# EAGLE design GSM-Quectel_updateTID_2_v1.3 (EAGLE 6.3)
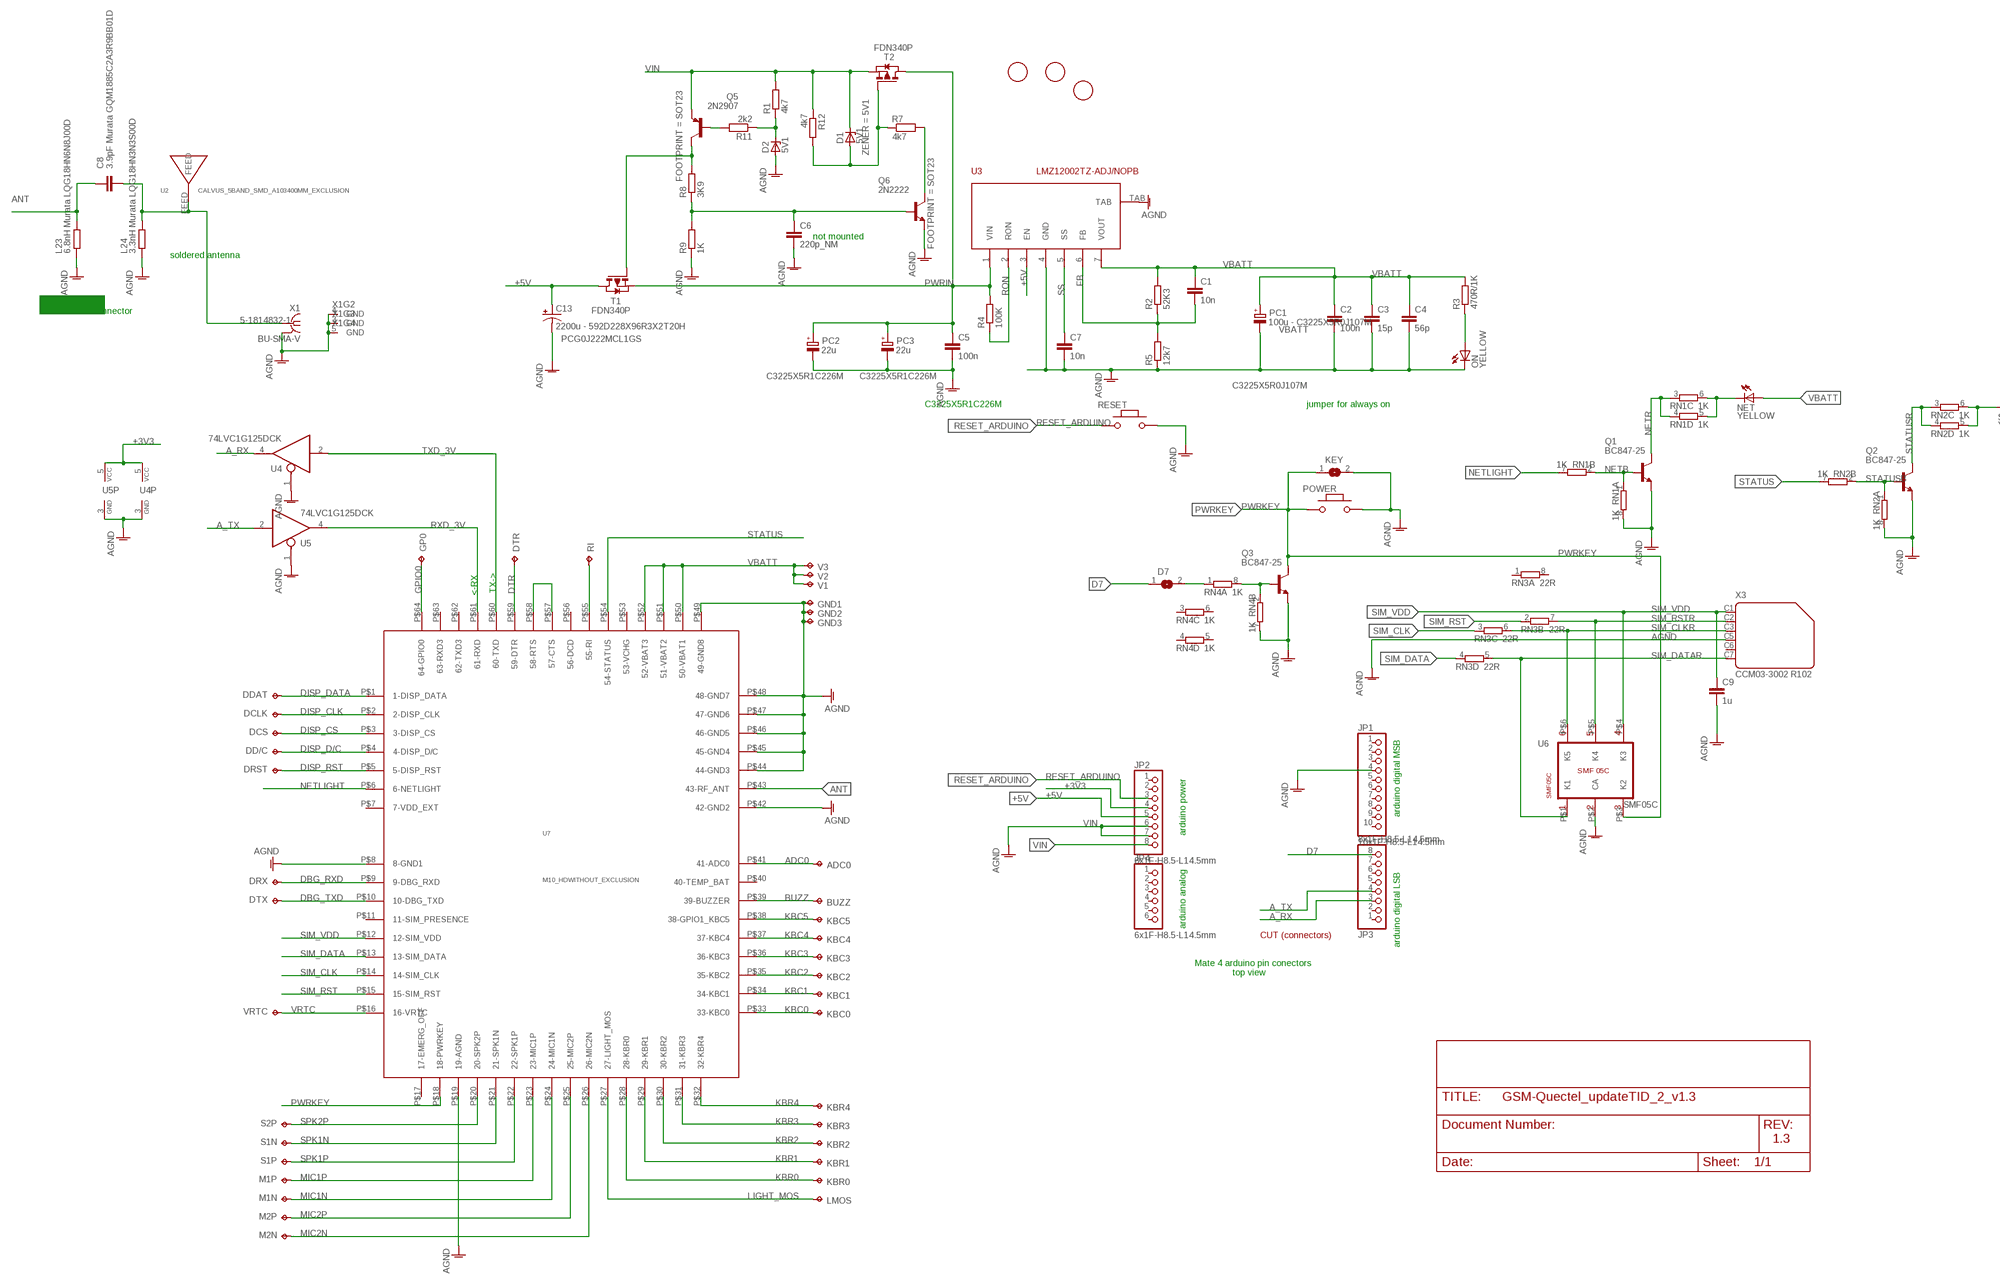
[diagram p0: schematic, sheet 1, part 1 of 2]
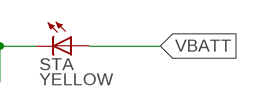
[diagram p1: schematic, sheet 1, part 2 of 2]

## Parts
ADC0  TPPAD1-09  [P1-09]
BUZZ  TPPAD1-09  [P1-09]
C1  10n  C-EU0603-RND  [C0603-ROUND]
C2  100n  C-EU0603-RND  [C0603-ROUND]
C3  15p  C-EU0603-RND  [C0603-ROUND]
C4  56p  C-EU0603-RND  [C0603-ROUND]
C5  100n  C-EU0603-RND  [C0603-ROUND]
C6  220p_NM  C-EU0603-RND  [C0603-ROUND]
C7  10n  C-EU0603-RND  [C0603-ROUND]
C8  3.9pF Murata GQM1885C2A3R9BB01D  C-EU0603-RND  [C0603-ROUND]
C9  1u  C-EU0603-RND  [C0603-ROUND]
C13  2200u - 592D228X96R3X2T20H  CPOL-US085CS-1AW  [085CS_1AW]
D1  5V1  ZENER-DIODESMB  [SMB]
D2  5V1  ZENER-DIODESMB  [SMB]
D7  SJ  [SJ]
DCLK  TPPAD1-09  [P1-09]
DCS  TPPAD1-09  [P1-09]
DD/C  TPPAD1-09  [P1-09]
DDAT  TPPAD1-09  [P1-09]
DRST  TPPAD1-09  [P1-09]
DRX  TPPAD1-09  [P1-09]
DTR  TPPAD1-09  [P1-09]
DTX  TPPAD1-09  [P1-09]
GND1  TPPAD1-09  [P1-09]
GND2  TPPAD1-09  [P1-09]
GND3  TPPAD1-09  [P1-09]
GP0  TPPAD1-09  [P1-09]
JP1  10x1F-H8.5-L14.5mm  PINHD-1X10TH  [1X10-TH]
JP2  8x1F-H8.5-L14.5mm  PINHD-1X8TH  [1X08-TH]
JP3  8x1F-H8.5-L14.5mm  PINHD-1X8TH  [1X08-TH]
JP4  6x1F-H8.5-L14.5mm  PINHD-1X6TH  [1X06-TH]
KBC0  TPPAD1-09  [P1-09]
KBC1  TPPAD1-09  [P1-09]
KBC2  TPPAD1-09  [P1-09]
KBC3  TPPAD1-09  [P1-09]
KBC4  TPPAD1-09  [P1-09]
KBC5  TPPAD1-09  [P1-09]
KBR0  TPPAD1-09  [P1-09]
KBR1  TPPAD1-09  [P1-09]
KBR2  TPPAD1-09  [P1-09]
KBR3  TPPAD1-09  [P1-09]
KBR4  TPPAD1-09  [P1-09]
KEY  SJ  [SJ]
L23  6.8nH Murata LQG18HN6N8J00D  R-EU_0603-RND  [R0603-ROUND]
L24  3.3nH Murata LQG18HN3N3S00D  R-EU_0603-RND  [R0603-ROUND]
LMOS  TPPAD1-09  [P1-09]
M1N  TPPAD1-09  [P1-09]
M1P  TPPAD1-09  [P1-09]
M2N  TPPAD1-09  [P1-09]
M2P  TPPAD1-09  [P1-09]
NET  YELLOW  LEDCHIP-LED0805  [CHIP-LED0805]
ON  YELLOW  LEDCHIP-LED0805  [CHIP-LED0805]
PC1  100u - C3225X5R0J107M  CPOL-EUSMCB  [SMC_B]
PC2  22u  CPOL-EUSMCB  [SMC_B]
PC3  22u  CPOL-EUSMCB  [SMC_B]
POWER  MYSMD_PB157  [SMD_157SW]
Q1  BC847-25  BC817-25SMD  [SOT23-BEC]
Q2  BC847-25  BC817-25SMD  [SOT23-BEC]
Q3  BC847-25  BC817-25SMD  [SOT23-BEC]
Q5  2N2907  MMBT2907ALT1-PNP-SOT23-BEC  [SOT23-BEC]
Q6  2N2222  MMBT2222ALT1-NPN-SOT23-BEC  [SOT23-BEC]
R1  4k7  R-EU_0603-RND  [R0603-ROUND]
R2  52K3  R-EU_0603-RND  [R0603-ROUND]
R3  470R/1K  R-EU_0603-RND  [R0603-ROUND]
R4  100K  R-EU_0603-RND  [R0603-ROUND]
R5  12k7  R-EU_0603-RND  [R0603-ROUND]
R7  4k7  R-EU_0603-RND  [R0603-ROUND]
R8  3K9  R-EU_0603-RND  [R0603-ROUND]
R9  1K  R-EU_0603-RND  [R0603-ROUND]
R11  2k2  R-EU_0603-RND  [R0603-ROUND]
R12  4k7  R-EU_0603-RND  [R0603-ROUND]
RESET  MYSMD_PB157  [SMD_157SW]
RI  TPPAD1-09  [P1-09]
RN1  1K  4R-NCAY16  [CAY16]
RN2  1K  4R-NCAY16  [CAY16]
RN3  22R  4R-NCAY16  [CAY16]
RN4  1K  4R-NCAY16  [CAY16]
S1N  TPPAD1-09  [P1-09]
S1P  TPPAD1-09  [P1-09]
S2P  TPPAD1-09  [P1-09]
STA  YELLOW  LEDCHIP-LED0805  [CHIP-LED0805]
T1  FDN340P  PMOSSOT23  [SOT-23]
T2  FDN340P  PMOSSOT23  [SOT-23]
U2  CALVUS_5BAND_SMD_A103400MM_EXCLUSION  [CALVUS_5BAND_SMD_A10340_0MM_EXCLUSION]
U3  LMZ12002TZ-ADJ/NOPB  LMZ1200X  [TZA-7]
U4  74LVC1G125DCK  [SC70-5]
U5  74LVC1G125DCK  [SC70-5]
U6  SMF05C  [SC70_6L]
U7  M10_HDWITHOUT_EXCLUSION  [M10_HD_WITHOUT_EXCLUSION]
U$1  FIDUCIALMOUNT  [FIDUCIA-MOUNT]
U$2  FIDUCIALMOUNT  [FIDUCIA-MOUNT]
U$3  FIDUCIALMOUNT  [FIDUCIA-MOUNT]
V1  TPPAD1-09  [P1-09]
V2  TPPAD1-09  [P1-09]
V3  TPPAD1-09  [P1-09]
VRTC  TPPAD1-09  [P1-09]
X1  BU-SMA-V  [BU-SMA-V]
X3  CCM03-3002 R102  CON-AMPHENOL_SIMLOCK-C707_10M006_512_2  [CON-AMPHENOL_C707_10M006_512_2]

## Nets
+3V3: JP2.4 U4.5(VCC) U5.5(VCC)
+5V: C13.+ JP2.5 T1.1(D) U3.3(EN)
A_RX: JP3.3 U4.4(O)
A_TX: JP3.4 U5.2(I)
ADC0: ADC0.TP U7.P$41(41-ADC0)
AGND: C2.2 C3.2 C4.2 C5.2 C6.2 C7.2 C9.2 C13.- D2.A GND1.TP GND2.TP GND3.TP JP1.4 JP2.6 JP2.7 KEY.2 L23.1 L24.1 ON.C PC1.- PC2.- PC3.- POWER.2 Q1.E Q2.E Q3.E Q6.E R5.1 R9.1 RESET.2 RN1.8 RN2.8 RN4.7 U3.4(GND) U3.TAB U4.1(OE) U4.3(GND) U5.1(OE) U5.3(GND) U6.P$2(CA) U7.P$8(8-GND1) U7.P$19(19-AGND) U7.P$42(42-GND2) U7.P$44(44-GND3) U7.P$45(45-GND4) U7.P$46(46-GND5) U7.P$47(47-GND6) U7.P$48(48-GND7) U7.P$49(49-GND8) X1.2(GND) X1.3(GND) X1.4(GND) X1.5(GND) X3.C5
ANT [antenna]: C8.1 L23.2 U7.P$43(43-RF_ANT)
ANTENA [antenna]: C8.2 L24.2 U2.FEED X1.1
BUZZ: BUZZ.TP U7.P$39(39-BUZZER)
D7: D7.1 JP3.8
DBG_RXD: DRX.TP U7.P$9(9-DBG_RXD)
DBG_TXD: DTX.TP U7.P$10(10-DBG_TXD)
DISP_CLK: DCLK.TP U7.P$2(2-DISP_CLK)
DISP_CS: DCS.TP U7.P$3(3-DISP_CS)
DISP_D/C: DD/C.TP U7.P$4(4-DISP_D/C)
DISP_DATA: DDAT.TP U7.P$1(1-DISP_DATA)
DISP_RST: DRST.TP U7.P$5(5-DISP_RST)
DTR: DTR.TP U7.P$59(59-DTR)
FB: C1.2 R2.1 R5.2 U3.6(FB)
GPIO0: GP0.TP U7.P$64(64-GPIO0)
KBC0: KBC0.TP U7.P$33(33-KBC0)
KBC1: KBC1.TP U7.P$34(34-KBC1)
KBC2: KBC2.TP U7.P$35(35-KBC2)
KBC3: KBC3.TP U7.P$36(36-KBC3)
KBC4: KBC4.TP U7.P$37(37-KBC4)
KBC5: KBC5.TP U7.P$38(38-GPIO1_KBC5)
KBR0: KBR0.TP U7.P$28(28-KBR0)
KBR1: KBR1.TP U7.P$29(29-KBR1)
KBR2: KBR2.TP U7.P$30(30-KBR2)
KBR3: KBR3.TP U7.P$31(31-KBR3)
KBR4: KBR4.TP U7.P$32(32-KBR4)
LIGHT_MOS: LMOS.TP U7.P$27(27-LIGHT_MOS)
MIC1N: M1N.TP U7.P$24(24-MIC1N)
MIC1P: M1P.TP U7.P$23(23-MIC1P)
MIC2N: M2N.TP U7.P$26(26-MIC2N)
MIC2P: M2P.TP U7.P$25(25-MIC2P)
N$1: U7.P$57(57-CTS) U7.P$58(58-RTS)
N$2: RI.TP U7.P$55(55-RI)
N$3: ON.A R3.1
N$4: Q3.B RN4.2 RN4.8
N$7: D7.2 RN4.1
N$8: Q6.C R7.2
N$9: Q5.C R8.2 T1.3(G)
N$10: Q5.B R11.2
N$11: C6.1 Q6.B R8.1 R9.2
N$13: D1.A R7.1 R12.2 T2.3(G)
N$14: D2.C R1.1 R11.1
NETB: Q1.B RN1.1 RN1.2
NETL: NET.C RN1.5 RN1.6
NETLIGHT: RN1.7 U7.P$6(6-NETLIGHT)
NETR: Q1.C RN1.3 RN1.4
PWRIN: C5.1 PC2.+ PC3.+ R4.2 T1.2(S) T2.1(D) U3.1(VIN)
PWRKEY: KEY.1 POWER.1 Q3.C U6.P$3(K2) U7.P$18(18-PWRKEY)
RESET_ARDUINO: JP2.3 RESET.1
RON: R4.1 U3.2(RON)
RXD_3V: U5.4(O) U7.P$61(61-RXD)
SIM_CLK: RN3.3 U7.P$14(14-SIM_CLK)
SIM_CLKR: RN3.6 U6.P$6(K5) X3.C3
SIM_DATA: RN3.4 U7.P$13(13-SIM_DATA)
SIM_DATAR: RN3.5 U6.P$1(K1) X3.C7
SIM_RST: RN3.2 U7.P$15(15-SIM_RST)
SIM_RSTR: RN3.7 U6.P$5(K4) X3.C2
SIM_VDD: C9.1 U6.P$4(K3) U7.P$12(12-SIM_VDD) X3.C1
SPK1N: S1N.TP U7.P$21(21-SPK1N)
SPK1P: S1P.TP U7.P$22(22-SPK1P)
SPK2P: S2P.TP U7.P$20(20-SPK2P)
SS: C7.1 U3.5(SS)
STATUS: RN2.7 U7.P$54(54-STATUS)
STATUSB: Q2.B RN2.1 RN2.2
STATUSL: RN2.5 RN2.6 STA.C
STATUSR: Q2.C RN2.3 RN2.4
TXD_3V: U4.2(I) U7.P$60(60-TXD)
VBATT: C1.1 C2.1 C3.1 C4.1 NET.A PC1.+ R2.2 R3.2 STA.A U3.7(VOUT) U7.P$50(50-VBAT1) U7.P$51(51-VBAT2) U7.P$52(52-VBAT3) V1.TP V2.TP V3.TP
VIN: D1.C JP2.8 Q5.E R1.2 R12.1 T2.2(S)
VRTC: U7.P$16(16-VRTC) VRTC.TP
Unconnected: JP1.1 JP1.2 JP1.3 JP1.5 JP1.6 JP1.7 JP1.8 JP1.9 JP1.10 JP2.1 JP2.2 JP3.1 JP3.2 JP3.5 JP3.6 JP3.7 JP4.1 JP4.2 JP4.3 JP4.4 JP4.5 JP4.6 RN3.1 RN3.8 RN4.3 RN4.4 RN4.5 RN4.6 U7.P$7(7-VDD_EXT) U7.P$11(11-SIM_PRESENCE) U7.P$17(17-EMERG_OFF) U7.P$40(40-TEMP_BAT) U7.P$53(53-VCHG) U7.P$56(56-DCD) U7.P$62(62-TXD3) U7.P$63(63-RXD3) X3.C6

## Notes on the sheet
- not mounted
- soldered antenna
- SMA or U.FL connector
- PCG0J222MCL1GS
- C3225X5R1C226M | jumper for always on
- <-RX
- TX->
- SMF05C
- arduino digital MSB
- arduino power
- arduino analog
- CUT (connectors)
- arduino digital LSB
- Mate 4 arduino pin conectors
- top view
- 1.3

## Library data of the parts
ADC0 BUZZ DCLK DCS DD/C DDAT DRST DRX DTR DTX GND1-GND3 GP0 KBC0 KBC1-KBC5 KBR0 KBR1-KBR4 LMOS M1N M1P M2N M2P RI S1N S1P S2P V1-V3 VRTC = testpad:TP: Test pad
C1-C9 = SmartPrj:C-EU: CAPACITOR, European symbol
C13 = rcl:CPOL-US: POLARIZED CAPACITOR, American symbol
D1 = diode:ZENER-DIODE: Z-Diode; ZENER: 5V1
D2 = diode:ZENER-DIODE: Z-Diode
D7 KEY = jumper:SJ: SMD solder JUMPER
JP1 = SmartPrj:PINHD-1X10: PIN HEADER
JP2 JP3 = SmartPrj:PINHD-1X8: PIN HEADER
JP4 = SmartPrj:PINHD-1X6: PIN HEADER
L23 L24 R1-R5 R7-R9 R11 R12 = SmartPrj:R-EU_: RESISTOR, European symbol
NET ON STA = led:LED: LED
PC1 = rcl:CPOL-EU: POLARIZED CAPACITOR, European symbol; PN: C3225X5R0J107M
PC2 PC3 = rcl:CPOL-EU: POLARIZED CAPACITOR, European symbol; PN: C3225X5R1C226M
POWER RESET = SmartPrj:MYSMD_PB157
Q1-Q3 = transistor-npn:BC817*: NPN Transistor
Q5 = transistor-neu-to92:*-PNP-: PNP Transistror; FOOTPRINT: SOT23
Q6 = transistor-neu-to92:*-NPN-: NPN Transistror; FOOTPRINT: SOT23
RN1-RN4 = resistor-dil:4R-N: Array Chip Resistor Source: RS Component / Phycomp
T1 T2 = zetex:PMOSSOT23: MOS FET
U2 = SmartPrj:CALVUS_5BAND_SMD_A10340
U3 = SmartPrj:LMZ1200X
U4 U5 = 74xx-little-us:74*1G125: Single Bus Buffer Gate with 3-State Output
U6 = SmartPrj:SMF05C: SMF05C-TVS Diode Array For ESD and Latch-Up Protection
U7 = GSM:M10_HD
U$1-U$3 = SmartPrj:FIDUCIALMOUNT
X1 = con-coax:BU-SMA-V: FEMALE SMA CONNECTOR Radiall distributor RS 112-3794; PN: 5-1814832-1
X3 = SmartPrj:CON-AMPHENOL_SIMLOCK-C707_10M006_512_2: C707A SIMLOCK® 2.5 mm with wide solder tails Source: Data sheet; OC_FARNELL: 1463072; OC_NEWARK: unknown

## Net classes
1 power: width 0.305 mm, drill 0.406 mm, clearance 0.178 mm
2 gnd: width 0.305 mm, drill 0.406 mm, clearance 0.178 mm
3 power usb: width 0.508 mm, drill 0.406 mm, clearance 0.178 mm
4 antenna: clearance 0.61 mm

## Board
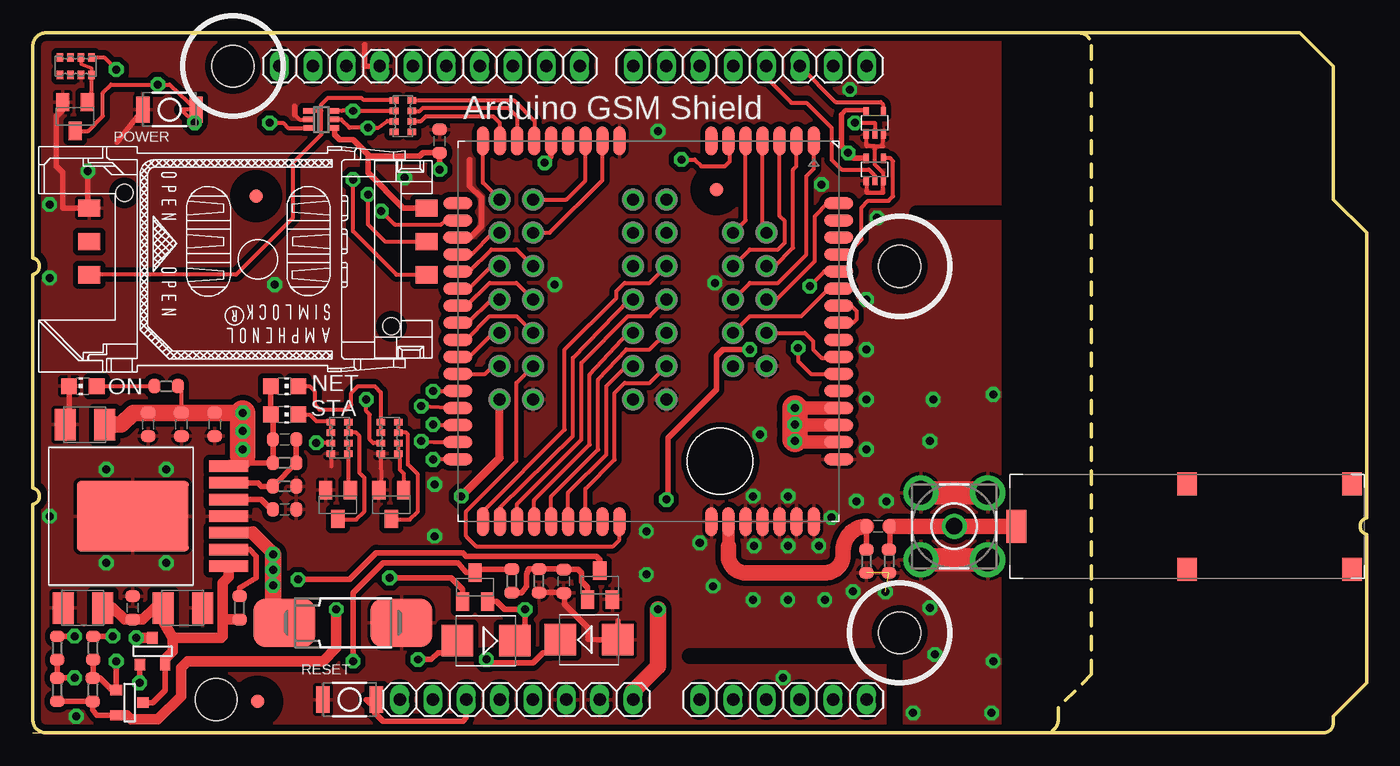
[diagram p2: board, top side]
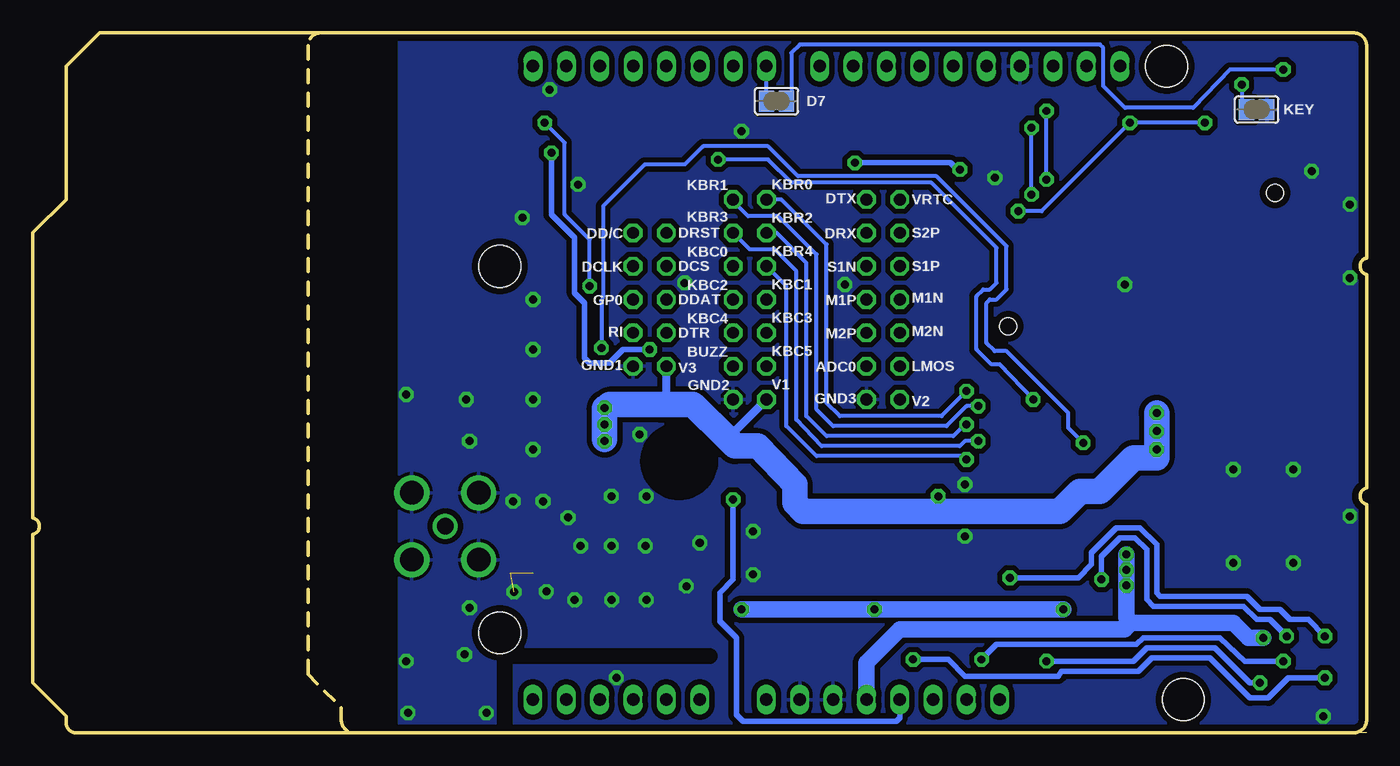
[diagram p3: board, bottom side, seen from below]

Size 101.6 x 53.34 mm. Coordinates in mm from the lower left corner, seen from the top.
Outline: 0,0 77.09,0
Outline: 77.11,0 arc90 78.11,1 78.11,1.91 80.64,4.45 80.64,52.34 arc90 79.64,53.34
Outline: 77.11,0 77.09,0
Outline: 77.09,0 1,0 arc-90 0,1 0,17.4 arc155 0,18.67 0,34.92 arc155 0,36.2 0,52.34 arc-90 1,53.34 79.64,53.34
Outline: 77.11,0 98.3,0 arc90 99.06,0.76 99.06,1.27 101.6,3.81 101.6,15.11 arc-155 101.6,16.38 101.6,38.1 99.06,40.64 99.06,50.8 96.52,53.34 79.64,53.34
Copper layers (1*16): Top 0.035mm / dielectric 1.5mm / Bottom 0.035mm
Design rules "default": minimum track width 10mil, minimum drill 22mil, track to track 8mil, track to pad 8mil, pad to pad 8mil, via to via 10mil, smd to smd 8mil, copper to edge 20mil, drill to drill 12mil, minimum pad ring 10mil, minimum via ring 10mil, stop-mask expansion 1mil, vias tented up to drill 30mil, thermal gap 10mil
Holes 3.2 mm at 66.04,35.56 66.04,7.62 15.24,50.8 13.97,2.54
tRestrict: area 74.9,16.6 to 76.8,18.4; 4 lines
bRestrict: 2 lines

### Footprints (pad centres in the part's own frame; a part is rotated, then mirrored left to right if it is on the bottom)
P1-09 = drill 0.9 pad 1.422 octagon: TP 0,0
C0603-ROUND = smd 0.898 x 1.1: 1 -0.889,0; 2 0.889,0
085CS_1AW = smd 4.7 x 3.7: + 4.45,0; - -4.45,0
SMB = smd 2.4 x 2.4: A 2.2,0; C -2.2,0
SJ = smd 1.168 x 1.6: 1 -0.762,0; 2 0.762,0
1X10-TH = drill 0.95 pad 1.422 long: 1 -11.43,0; 2 -8.89,0; 3 -6.35,0; 4 -3.81,0; 5 -1.27,0; 6 1.27,0; 7 3.81,0; 8 6.35,0; 9 8.89,0; 10 11.43,0
1X08-TH = drill 0.95 pad 1.422 long: 1 -8.89,0; 2 -6.35,0; 3 -3.81,0; 4 -1.27,0; 5 1.27,0; 6 3.81,0; 7 6.35,0; 8 8.89,0
1X06-TH = drill 0.95 pad 1.422 long: 1 -6.35,0; 2 -3.81,0; 3 -1.27,0; 4 1.27,0; 5 3.81,0; 6 6.35,0
R0603-ROUND = smd 0.898 x 1.1: 1 -0.889,0; 2 0.889,0
CHIP-LED0805 = smd 1.2 x 1.2: A 0,-1.05; C 0,1.05
SMC_B = smd 1.6 x 2.4: + -1.5,0; - 1.5,0
SMD_157SW = smd 1.016 x 1.981: 1 -2.032,0; 2 2.032,0
SOT23-BEC = smd 1 x 1.4: B -0.95,-1.1; C 0,1.1; E 0.95,-1.1
CAY16 = smd 0.5 x 0.65: 1 -1.2,-0.675; 2 -0.4,-0.675; 3 0.4,-0.675; 4 1.2,-0.675; 5 1.2,0.675; 6 0.4,0.675; 7 -0.4,0.675; 8 -1.2,0.675
SOT-23 = smd 0.787 x 0.889: 1 0.025,-1.016; 2 -0.94,1.016; 3 0.991,1.016
CALVUS_5BAND_SMD_A10340_0MM_EXCLUSION = smd 2.5 x 1.5: FEED 3.95,0.5 | smd 1.75 x 1.5: FIXINGPOINT$1 0.7,26.05; FIXINGPOINT$2 7.22,26.05; FIXINGPOINT$3 0.7,13.49; FIXINGPOINT$4 7.22,13.49
TZA-7 = smd 0.89 x 3.06: 1 -3.81,-7.305; 2 -2.54,-7.305; 3 -1.27,-7.305; 4 0,-7.305; 5 1.27,-7.305; 6 2.54,-7.305; 7 3.81,-7.305 | smd 5.35 x 8.54: TAB 0,0
SC70-5 = smd 0.4 x 0.7: 1 -0.65,-0.85; 2 0,-0.85; 3 0.65,-0.85; 4 0.65,0.85; 5 -0.65,0.85
SC70_6L = smd 0.4 x 0.85: P$1 -0.65,-0.94; P$2 0,-0.94; P$3 0.65,-0.935; P$4 0.65,0.94; P$5 0,0.94; P$6 -0.65,0.94
M10_HD_WITHOUT_EXCLUSION = smd 2.2 x 0.9: P$1 0,27.1; P$2 0,25.8; P$3 0,24.5; P$4 0,23.2; P$5 0,21.9; P$6 0,20.6; P$7 0,19.3; P$8 0,12.3; P$9 0,11; P$10 0,9.7; P$11 0,8.4; P$12 0,7.1; P$13 0,5.8; P$14 0,4.5; P$15 0,3.2; P$16 0,1.9; P$33 29,1.9; P$34 29,3.2; P$35 29,4.5; P$36 29,5.8; P$37 29,7.1; P$38 29,8.4; P$39 29,9.7; P$40 29,11; P$41 29,12.3; P$42 29,19.3; P$43 29,20.6; P$44 29,21.9; P$45 29,23.2; P$46 29,24.5; P$47 29,25.8; P$48 29,27.1 | smd 0.9 x 2.2: P$17 4.75,0; P$18 6.05,0; P$19 7.35,0; P$20 8.65,0; P$21 9.95,0; P$22 11.25,0; P$23 12.55,0; P$24 13.85,0; P$25 15.15,0; P$26 16.45,0; P$27 17.75,0; P$28 19.05,0; P$29 20.35,0; P$30 21.65,0; P$31 22.95,0; P$32 24.25,0; P$49 24.25,29; P$50 22.95,29; P$51 21.65,29; P$52 20.35,29; P$53 19.05,29; P$54 17.75,29; P$55 16.45,29; P$56 15.15,29; P$57 13.85,29; P$58 12.55,29; P$59 11.25,29; P$60 9.95,29; P$61 8.65,29; P$62 7.35,29; P$63 6.05,29; P$64 4.75,29
FIDUCIA-MOUNT = smd 1.016 x 1.016: P$1 0,0
BU-SMA-V = drill 1.27: 1 0,0 | drill 1.778: 2 -2.55,2.55; 3 2.55,2.55; 4 2.55,-2.55; 5 -2.55,-2.55
CON-AMPHENOL_C707_10M006_512_2 = smd 1.7 x 1.3: C1 -12.85,-3.915; C2 -12.85,-1.375; C3 -12.85,1.165; C5 12.85,-3.915; C6 12.85,-1.375; C7 12.85,1.165 | hole 1.3: 10.16,-5.08; -10.16,5.08

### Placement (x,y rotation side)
ADC0  38.1,27.94 0 top
BUZZ  48.26,27.94 0 top
C1  19.18,22.35 0 top
C2  8.78,23.5 270 top
C3  13.86,23.5 270 top
C4  11.32,23.5 270 top
C5  7.62,9.53 90 top
C6  40.44,11.55 270 top
C7  19.18,17.02 0 top
C8  64.39,15.75 0 top
C9  30.99,45.09 90 top
C13  23.62,8.38 180 top
D1  34.52,7.03 180 top
D2  42.37,7.1 0 top
D7  44.96,48.13 0 bottom
DCLK  55.88,35.56 0 top
DCS  53.34,35.56 0 top
DD/C  55.88,38.1 0 top
DDAT  53.34,33.02 0 top
DRST  53.34,38.1 0 top
DRX  38.1,38.1 0 top
DTR  53.34,30.48 0 top
DTX  38.1,40.64 0 top
GND1  55.88,27.94 0 top
GND2  48.26,25.4 0 top
GND3  38.1,25.4 0 top
GP0  55.88,33.02 0 top
JP1  30.23,50.8 0 top
JP2  36.83,2.54 0 top
JP3  54.61,50.8 180 top
JP4  57.15,2.54 0 top
KBC0  48.26,35.56 0 top
KBC1  45.72,33.02 0 top
KBC2  48.26,33.02 0 top
KBC3  45.72,30.48 0 top
KBC4  48.26,30.48 0 top
KBC5  45.72,27.94 0 top
KBR0  45.72,40.64 0 top
KBR1  48.26,40.64 0 top
KBR2  45.72,38.1 0 top
KBR3  48.26,38.1 0 top
KBR4  45.72,35.56 0 top
KEY  8.38,47.5 0 bottom
L23  63.5,13.08 90 top
L24  65.23,13.08 90 top
LMOS  35.56,27.94 0 top
M1N  35.56,33.02 0 top
M1P  38.1,33.02 0 top
M2N  35.56,30.48 0 top
M2P  38.1,30.48 0 top
NET  19.18,26.42 270 top
ON  3.81,26.42 90 top
PC1  3.97,23.5 180 top
PC2  11.43,9.53 0 top
PC3  3.81,9.53 180 top
POWER  10.41,47.5 180 top
Q1  27.3,17.4 180 top
Q2  23.24,17.4 180 top
Q3  3.22,46.96 180 top
Q5  33.69,11.11 0 top
Q6  43.19,11.27 0 top
R1  1.85,3.29 270 top
R2  19.18,20.57 180 top
R3  10.16,26.42 0 top
R4  15.75,9.53 270 top
R5  19.18,18.8 180 top
R7  4.59,6.47 90 top
R8  36.48,11.58 90 top
R9  38.54,11.59 90 top
R11  1.86,6.46 90 top
R12  4.57,3.28 90 top
RESET  24.13,2.54 180 top
RI  55.88,30.48 0 top
RN1  27.18,22.48 90 top
RN2  23.37,22.48 90 top
RN3  28.19,46.99 90 top
RN4  3.27,50.8 180 top
S1N  38.1,35.56 0 top
S1P  35.56,35.56 0 top
S2P  35.56,38.1 0 top
STA  19.18,24.26 270 top
T1  9.14,6.22 180 top
T2  7.37,2.28 90 top
U2  74.42,19.68 270 top
U3  7.62,16.51 90 top
U4  64.14,46.48 0 top
U5  64.14,42.93 0 top
U6  21.97,46.74 270 top
U7  32.38,45.1 270 top
U$1  17.02,40.89 0 top
U$2  52.07,41.4 0 top
U$3  17.11,2.4 0 top
V1  45.72,25.4 0 top
V2  35.56,25.4 0 top
V3  53.34,27.94 0 top
VRTC  35.56,40.64 0 top
X1  70.18,15.75 0 top
X3  17.14,36.07 180 top

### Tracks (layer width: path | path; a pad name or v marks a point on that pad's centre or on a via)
+3V3  (via drill 0.61)
  Top 0.356: 61.59,47.12 61.91,47.43 63.48,47.43
  Top 0.406: 61.59,47.12 61.59,44.7 v62.1,44.2 62.52,43.78 U5.5 | v48.26,17.78 48.39,17.91 48.39,22.48 52.07,26.16 52.07,28.7 52.58,29.21 v54.61,29.21 | 63.48,47.43 U4.5
  Bottom 0.406: v62.1,44.2 62.1,39.5 60.33,37.72 60.33,33.53 59.56,32.77 59.56,28.57 59.18,28.19 57.66,28.19 56.64,29.21 v54.61,29.21 | v48.26,17.78 48.26,11.68 49.28,10.67 49.28,8.51 48.01,7.24 48.01,1.4 47.5,0.89 35.81,0.89 35.56,1.14 JP2.4
+5V  (via drill 0.61)
  Top 0.813: T1.1 v7.87,7.24
  Top 0.914: 16.76,15.24 U3.3
  Top 1.016: 16.76,15.24 18.16,13.84 v18.29,13.61
  Top 1.27: v18.29,13.61 v18.29,12.42 18.29,8 18.41,7.87 18.66,7.87 | 18.66,7.87 C13.+ | 18.66,7.87 18.67,7.87 C13.+
  Bottom 1.27: v18.29,13.61 v18.29,11.23 18.29,8.76 17.91,8.38 | v7.87,7.24 9.02,7.24 10.16,8.38 17.91,8.38 | 17.91,8.38 18.41,7.87 35.56,7.87 38.1,5.33 JP2.5
A_RX
  Top 0.305: U4.4 64.78,47.86 64.58,48.07 61.15,48.07 JP3.3
A_TX
  Top 0.305: U5.2 64.14,42.47 63.68,42.93 61.59,42.93 60.83,43.69 60.83,46.1 58.93,48.01 57.78,48.01 55.88,49.91 JP3.4
ADC0
  Top 0.305: U7.P$41 44.69,14.71 44.2,14.22 33.78,14.22 33.02,14.99 33.02,16.89 36.83,20.7 36.83,26.67 ADC0.TP
AGND  (via drill 0.61, 0.61 pad 0.81)  (2 unrouted)
  Top 0.305: 64.14,44.7 64.77,44.7 64.77,45.62 U4.3 | U5.1 63.48,41.29 63.5,41.15 64.77,41.15 64.77,42.06 U5.3 64.78,42.66 64.14,43.31 64.14,44.7 | RN1.8 26.63,17.97 Q1.E | 64.14,44.7 63.5,44.7 63.5,45.62 U4.1 | Q3.E 2.46,48.56 | RN4.7 3.68,50.11 | RN2.8 arc90 22.73,21.19 22.73,20.32 | U6.P$2 20.32,46.74 19.94,47.12
  Top 0.406: U7.P$19 33.3,37.75 34.16,38.61 34.16,40.77 33.27,41.66 33.27,43.69 | 6.41,45.02 POWER.2 | v4.19,42.8 4.19,40.09 X3.C5 2.27,39.98 2.29,42.67 1.78,43.18 1.78,46.99 2.27,47.48 Q3.E | ON.C 2.76,23.84 PC1.- | R9.1 40.4,10.7 C6.2 40.51,10.59 40.51,9.78 42.29,8 42.29,7.11 43.06,7.1 D2.A 44.56,8.52 | 44.2,10.11 Q6.E | JP1.4 25.27,50.8 25.27,52.45 | 19.94,47.12 19.94,47.75
  Top 1.778: X1.5 X1.4 | X1.2 X1.3
  other vias: 54.94,14.25 57.53,14.25 60.83,16.41 59.87,14.25 54.86,10.13 57.51,10.13 60.33,10.13 62.48,10.77 50.8,14.48 51.82,11.18 62.74,17.65 73.15,5.46 68.33,9.53 64.95,10.74 67.06,1.52 73.03,1.52 68.33,22.23 46.74,12.06 60.07,41.78 63.5,21.59 63.5,25.4 63.5,29.21 63.5,33.02 64.31,39.24 62.23,49.02 1.27,40.26 1.27,34.67 3.3,1.27 1.27,16.51 30.61,18.92 30.61,14.99 46.74,15.37 54.86,18.03 57.53,18.03 55.37,22.73 57.15,4.19 10.16,20.07 5.59,20.07 5.59,12.95 10.16,12.95 18.41,34.16 47.62,45.85 39.75,34.16 51.94,34.29 28.32,42.29 65.02,17.65 68.58,25.4 73.15,25.78 68.71,5.97
  pour Bottom (isolate 0.406): -0.51,54.86 73.66,54.86 73.66,-0.38 -0.25,-0.25 -0.51,-0.25
  pour Top (isolate 0.406): -0.51,54.86 73.66,54.86 73.66,-0.38 -0.51,-0.38
ANT
  Top 0.406: C8.1 L23.2
  Top 0.965: 52.98,14.22 U7.P$43
  Top 1.168: 52.98,14.22 52.98,13.72 arc90 54.13,12.19 60.33,12.19 arc90 61.72,13.59 61.72,13.84 arc-90 C8.1
ANTENA
  Top 0.406: 65.53,15.53 C8.2 65.28,13.97 L24.2
  Top 1.168: U2.FEED arc90 74.78,15.75 X1.1 C8.2
BUZZ
  Top 0.305: U7.P$39 42.09,18.59 44.32,20.83 44.32,25.91 45.09,26.67 46.99,26.67 BUZZ.TP
D7
  Bottom 0.305: D7.1 JP3.8
DBG_RXD
  Top 0.305: U7.P$9 43.38,42.12 39.37,38.1 DRX.TP
DBG_TXD
  Top 0.305: U7.P$10 42.09,42.09 40.64,40.64 DTX.TP
DISP_CLK
  Top 0.305: DCLK.TP 56.52,35.56 57.91,36.96 57.91,42.93 58.17,43.18 58.17,45.08 U7.P$2
DISP_CS
  Top 0.305: U7.P$3 56.88,39.38 57.28,38.99 57.28,37.34 56.77,36.83 54.61,36.83 DCS.TP
DISP_D/C
  Top 0.305: U7.P$4 55.59,38.4 DD/C.TP
DISP_DATA
  Top 0.305: U7.P$1 59.48,42.98 58.93,42.42 58.93,36.45 56.77,34.29 54.61,34.29 DDAT.TP
DISP_RST
  Top 0.305: U7.P$5 54.28,39.05 DRST.TP
DTR
  Top 0.305: U7.P$59 60.65,33.85 58.55,31.75 54.61,31.75 DTR.TP
FB
  Top 0.406: U3.6 17.14,19.05 17.4,18.8 R5.2 R2.1 C1.2
GPIO0
  Top 0.305: GP0.TP 56.64,33.02 59.56,35.94 59.56,39.37 60.58,40.39 61.35,40.39 U7.P$64
KBC0
  Top 0.305: U7.P$33 34.28,16.89 40.51,23.11 40.51,29.21 44.45,33.15 44.45,33.66 45.09,34.29 46.99,34.29 KBC0.TP
KBC1
  Top 0.305: U7.P$34 35.59,17.17 41.15,22.61 41.15,28.57 45.47,33.02 KBC1.TP
KBC2
  Top 0.305: U7.P$35 36.88,17.45 41.78,22.35 41.78,28.19 45.34,31.75 46.99,31.75 KBC2.TP
KBC3
  Top 0.305: U7.P$36 38.19,17.74 42.42,21.97 42.42,27.3 45.34,30.48 KBC3.TP
KBC4
  Top 0.305: U7.P$37 39.48,18.02 43.05,21.59 43.05,26.92 45.21,29.21 46.99,29.21 KBC4.TP
KBC5
  Top 0.305: U7.P$38 40.78,18.31 43.69,21.21 43.69,26.42 45.21,27.94 KBC5.TP
KBR0  (via drill 0.61)
  Top 0.305: U7.P$28 32.37,26.04 v30.48,26.04
  Bottom 0.305: v30.48,26.04 32.38,24.13 40.13,24.13 41.15,25.15 41.15,37.21 44.58,40.64 KBR0.TP
KBR1  (via drill 0.61)
  Top 0.305: U7.P$29 32.37,24.77 v29.59,24.89
  Bottom 0.305: v29.59,24.89 30.48,24.89 32,23.37 40.64,23.37 41.91,24.64 41.91,36.45 44.83,39.37 47.12,39.37 48.26,40.51 KBR1.TP
KBR2  (via drill 0.61)
  Top 0.305: U7.P$30 30.52,23.45 v30.48,23.5
  Bottom 0.305: KBR2.TP 44.96,38.1 42.67,35.81 42.67,24.13 41.15,22.61 31.5,22.61 30.61,23.5 v30.48,23.5
KBR3  (via drill 0.61)
  Top 0.305: U7.P$31 30.55,22.15 v29.59,22.23
  Bottom 0.305: KBR3.TP 46.99,36.83 45.09,36.83 43.43,35.18 43.43,23.88 41.53,21.84 30.99,21.84 30.61,22.23 v29.59,22.23
KBR4  (via drill 0.61)
  Top 0.305: U7.P$32 30.63,20.85 v30.48,20.83
  Bottom 0.305: KBR4.TP 44.2,34.04 44.2,23.37 41.91,21.08 30.73,21.08 v30.48,20.83 30.63,20.85
LIGHT_MOS
  Top 0.305: U7.P$27 34.46,27.35 35.05,27.94 LMOS.TP
MIC1N
  Top 0.305: U7.P$24 33.16,31.25 34.92,33.02 M1N.TP
MIC1P
  Top 0.305: M1P.TP 36.83,34.29 34.8,34.29 33.06,32.55 U7.P$23
MIC2N
  Top 0.305: U7.P$26 33.22,28.65 35.05,30.48 M2N.TP
MIC2P
  Top 0.305: M2P.TP 36.83,31.75 34.8,31.75 33,29.95 U7.P$25
N$1
  Top 0.305: U7.P$58 62.32,32.55 62.74,32.13 62.74,31.5 62.48,31.24 61.39,31.24 U7.P$57
N$2
  Top 0.305: RI.TP 58.8,30.48 59.44,29.84 59.44,29.21 60.07,28.57 61.31,28.57 U7.P$55
N$3
  Top 0.305: ON.A R3.1
N$4
  Top 0.254: RN4.2 3.67,50.94 4.47,50.65 RN4.8
  Top 0.305: RN4.8 4.47,48.87 Q3.B
N$7  (via drill 0.61)
  Top 0.305: RN4.1 5.42,51.48 v6.35,50.55
  Bottom 0.305: D7.2 43.81,48.51 43.81,51.82 43.18,52.45 20.32,52.45 20.07,52.2 20.07,49.28 18.41,47.62 13.21,47.62 10.41,50.55 v6.35,50.55
N$8  (via drill 0.61)
  Top 0.406: Q6.C 43.19,13.2 42.93,13.46 33.02,13.46 32.77,13.72 26.16,13.72 24.13,11.68 v20.19,11.68 | v6.1,7.37 R7.2
  Bottom 0.406: v20.19,11.68 20.19,13.46 18.8,14.86 17.65,14.86 16.76,13.97 16.76,10.16 16.26,9.65 9.4,9.65 8.38,8.64 7.37,8.64 v6.1,7.37
N$9  (via drill 0.61)
  Top 0.406: T1.3 8.15,4.09 v8.13,3.81 | v24.38,5.46 24.38,10.67 26.67,12.95 32.4,12.95 33.01,12.21 Q5.C 33.69,12.47 R8.2
  Bottom 0.406: v8.13,3.81 8.89,3.81 11.56,6.48 16.76,6.48 17.78,5.46 v24.38,5.46
N$10  (via drill 0.6, 0.61)
  Top 0.406: v3.17,7.37 1.93,7.37 R11.2 | Q5.B 32.74,10.95 31.88,11.81 v27.18,11.81
  Bottom 0.406: v27.18,11.81 21.97,11.81 20.95,12.83 20.95,13.72 19.05,15.62 17.27,15.62 16,14.35 16,10.67 15.75,10.41 9.14,10.41 8.13,9.4 6.6,9.4 5.84,8.64 4.45,8.64 v3.17,7.37
N$11
  Top 0.406: R8.1 36.51,10.67 37.21,10.67 37.59,11.18 37.59,12.06 37.75,12.48 R9.2 40.4,12.48 C6.1 40.45,12.45 41.53,12.45 41.78,12.19 41.78,11.56 42.24,11.1 Q6.B
N$13  (via drill 0.6)
  Top 0.406: R7.1 4.59,4.17 R12.2 4.84,4.19 5.08,4.19 6,3.27 T2.3 v6.35,5.46 | v29.34,5.59 30.35,5.59 30.86,6.1 31.62,6.1 31.62,6.71 31.64,6.73 | 31.64,6.73 32.13,6.71 D1.A | 31.64,6.73 31.5,6.73
  Bottom 0.406: v29.34,5.59 28.19,6.73 17.53,6.73 17.02,7.24 11.18,7.24 9.27,5.46 v6.35,5.46
N$14  (via drill 0.61)
  Top 0.406: R1.1 1.86,4.18 | 1.86,4.18 1.86,4.15 1.91,4.19 v3.17,4.19 | v34.54,5.59 35.05,5.33 38.1,5.33 38.86,6.1 39.37,6.1 39.37,6.84 39.39,6.86 D2.C | 1.86,4.18 R11.1
  Bottom 0.406: v3.17,4.19 5.97,4.19 7.49,2.67 8.89,2.67 11.94,5.71 16.38,5.71 17.4,4.7 23.24,4.7 23.5,4.32 30.61,4.32 31.88,5.59 v34.54,5.59
NETB
  Top 0.305: RN1.2 RN1.1 27.94,21.24 27.94,20.07 28.25,19.75 Q1.B
NETL
  Top 0.305: RN1.6 RN1.5 26.5,25.95 26.04,26.42 24.77,26.42 24.26,25.91 24.26,25.02 23.88,24.64 21.84,24.64 21.46,25.02 21.46,26.04 21.08,26.42 NET.C
NETLIGHT  (via drill 0.61)
  Top 0.305: RN1.7 25.93,22.08 25.65,22.35 25.65,24.26 25.4,24.51 v25.4,25.4 | v49.4,43.69 50.42,43.69 50.93,43.18 52.7,43.18 53.09,43.56 53.09,44.32 52.96,44.45 52.96,45.07 U7.P$6
  Bottom 0.305: v25.4,25.4 27.94,28.07 28.57,28.07 29.72,29.21 29.72,33.27 29.21,33.78 28.7,33.78 28.19,34.29 28.19,36.96 33.15,41.91 43.81,41.91 45.59,43.69 v49.4,43.69
NETR
  Top 0.305: RN1.4 RN1.3 28.43,22.88 28.57,22.73 28.57,20.45 29.34,19.68 29.34,16.89 28.7,16.26 27.39,16.26 Q1.C
PWRIN
  Top 0.406: T1.2 10.08,3.23 9.14,2.29 8.4,2.29 T2.1
  Top 0.813: 10.67,7.24 9.93,8.48 PC2.+ 9.27,9.53 8.38,8.64 C5.1 6.99,8.64 6.1,9.53 PC3.+ | 10.67,7.24 10.67,6.22 10.08,5.64 T1.2 | U3.1 14.93,11.87 14.86,11.81 14.48,11.43 14.48,8.64 | 14.48,8.64 14.48,7.37 14.35,7.24 10.67,7.24 | 14.48,8.64 R4.2
PWRKEY  (via drill 0.6, 0.61)
  Top 0.305: U7.P$18 31.43,39.05 31.11,38.73 27.56,38.73 v26.54,39.75 | Q3.C 4.2,45.86 5.33,46.99 5.33,48.77 5.97,49.4 v9.53,49.4 10.41,49.4 POWER.1 11.3,47.5 v12.32,46.48 | U6.P$3 19.45,46.09 19.05,46.48 v18.03,46.48
  Bottom 0.305: v26.54,39.75 24.77,39.75 v18.03,46.48 v12.32,46.48 | v9.53,49.4 9.53,47.88 KEY.1
RESET_ARDUINO
  Top 0.406: RESET.1 25.4,2.54 26.04,1.91 26.04,1.52 26.67,0.89 32.77,0.89 33.02,1.14 JP2.3
RON
  Top 0.406: U3.2 16.51,13.97 17.02,13.46 17.02,11.81 15.75,11.05 R4.1
RXD_3V
  Top 0.305: U7.P$61 61.98,36.45 63.12,37.59 63.12,40.03 63.63,40.54 65.17,40.54 65.53,40.89 65.53,43.56 65.32,43.78 U5.4
SIM_CLK
  Top 0.305: U7.P$14 36.88,46.94 36.2,47.62 29.72,47.62 29.46,47.37 28.89,47.37 RN3.3
SIM_CLKR  (via drill 0.6, 0.61)
  Top 0.305: X3.C3 27.71,34.9 24.38,38.23 v24.38,42.16 | U6.P$6 23.55,47.39 v24.38,47.39 RN3.6
  Bottom 0.305: v24.38,42.16 v24.38,47.39
SIM_DATA
  Top 0.305: U7.P$13 38.23,45.14 38.23,46.61 36.65,48.19 RN3.4
SIM_DATAR
  Top 0.305: X3.C7 15.47,34.9 19.81,39.24 19.81,43.43 21.97,45.59 21.97,47.39 | 21.97,47.39 21.97,47.88 22.48,48.39 25.02,48.39 25.15,48.26 27.45,48.26 RN3.5 | 21.97,47.39 U6.P$1
SIM_RST
  Top 0.305: RN3.2 29.59,46.61 29.95,46.97 35.07,46.97 35.56,46.48 35.56,45.12 U7.P$15
SIM_RSTR  (via drill 0.61)
  Top 0.305: X3.C2 26.82,37.44 25.53,38.73 v25.53,41.02 | U6.P$5 23.5,46.74 24.13,46.1 v25.53,46.1 26.29,46.1 26.99,46.61 27.5,46.61 RN3.7
  Bottom 0.305: v25.53,41.02 v25.53,46.1
SIM_VDD  (via drill 0.61)
  Top 0.406: 25.53,44.07 25.65,43.94 29.46,43.94 29.72,44.2 C9.1 v30.99,42.93 | U7.P$12 39.48,43.93 v38.99,43.43 | X3.C1 28.22,39.98 25.53,42.67 25.53,44.07 | U6.P$4 22.99,46.01 22.99,45.59 23.37,45.21 24.38,45.21 25.53,44.07
  Bottom 0.406: v30.99,42.93 31.19,42.93 31.7,43.43 v38.99,43.43
SPK1N
  Top 0.305: S1N.TP 36.83,36.83 34.92,36.83 33.24,35.15 U7.P$21
SPK1P
  Top 0.305: U7.P$22 33.22,33.85 34.92,35.56 S1P.TP
SPK2P
  Top 0.305: U7.P$20 33.4,36.45 35.05,38.1 S2P.TP
SS
  Top 0.406: U3.5 17.4,17.78 18.16,17.02 C7.1
STATUS  (via drill 0.61)
  Top 0.305: RN2.7 21.61,22.08 v21.59,22.1 | U7.P$54 59.26,27.35 58.29,28.32 v58.29,29.34
  Bottom 0.305: v58.29,29.34 58.29,32.89 58.17,33.27 58.17,40.13 54.99,43.31 51.94,43.31 50.55,44.7 45.59,44.7 43.31,42.42 32.77,42.42 27.43,37.08 27.43,33.78 28.19,33.02 28.7,33.02 28.96,32.77 28.96,29.72 28.32,29.08 27.43,29.08 22.73,24.38 22.73,23.24 v21.59,22.1
STATUSB
  Top 0.305: RN2.2 RN2.1 24.04,18.65 Q2.B
  Top 0.406: Q2.B 24.42,18.5
STATUSL
  Top 0.305: RN2.6 RN2.5 22.75,23.75 21.59,23.75 21.08,24.26 STA.C
STATUSR
  Top 0.305: RN2.4 RN2.3 24.62,22.88 24.89,22.61 24.89,19.81 25.27,19.43 25.27,16.89 24.64,16.26 23.28,16.26 Q2.C
TXD_3V  (via drill 0.61)
  Top 0.305: v62.61,46.48 64.14,46.48 U4.2 | U7.P$60 60.3,35.15 v59.18,34.04
  Bottom 0.305: v62.61,46.48 61.09,44.96 61.09,39.5 59.18,37.59 v59.18,34.04
VBATT  (via drill 0.61)
  Top 0.305: C4.1 11.32,26.4 R3.2
  Top 0.406: NET.A STA.A 18.29,23.97 C1.1 R2.2 16.26,20.57 16,20.45
  Top 0.61: V2.TP 35.56,20.95 v32.64,18.03
  Top 0.914: U3.7 16,20.32 16,20.45
  Top 1.016: 16,21.08 16,20.45 | U7.P$50 58.24,22.15 58.04,22.35 | U7.P$51 58.08,23.45 v58.04,23.5 | U7.P$52 58.05,24.75 v58.04,24.77
  Top 1.27: v16,24.38 C3.1 C4.1 C2.1 7.63,24.38 6.74,23.5 PC1.+
  Top 1.93: v16,22.99 16,21.08 | v16,22.99 16,24.26 | v58.04,24.77 v58.04,23.5 58.04,22.35 | v16,24.38 v16,22.99
  Bottom 0.61: V3.TP 53.34,25.4 53.72,25.02 | 32.64,16.89 v32.64,18.03 | 58.04,22.35 v58.04,22.23 | 48.7,22.42 V1.TP
  Bottom 1.93: v16,24.38 v16,21.59 16,20.95 17.78,20.95 20.32,18.41 21.84,18.41 23.37,16.89 32.64,16.89 42.93,16.89 43.56,17.53 43.56,18.92 46.35,21.84 48.13,21.84 48.7,22.42 51.31,25.02 53.72,25.02 57.66,25.02 58.04,24.64 | 58.04,24.64 58.04,22.35 | 58.04,24.64 v58.04,24.77
VIN  (via drill 0.61)
  Top 0.406: R1.2 4.06,2.4 R12.1 4.57,1.88 4.57,1.78 4.88,1.34 T2.2 | 34.64,9.81 Q5.E 35.33,10.01 35.94,9.4 v37.49,9.4 37.49,6.78 D1.C 35.81,6.79
  Top 0.813: T2.2 7.17,1.34 7.49,1.04 9.53,1.04 11.3,2.79 11.3,4.95 11.81,5.46 22.1,5.46 23.11,6.48 v23.11,9.4
  Top 1.27: v47.62,9.4 47.62,5.08 45.72,3.17 JP2.8
  Bottom 1.27: v47.62,9.4 v37.49,9.4 v23.11,9.4
VRTC
  Top 0.305: U7.P$16 34.28,41.91 VRTC.TP

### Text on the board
tPlace: Arduino GSM Shield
